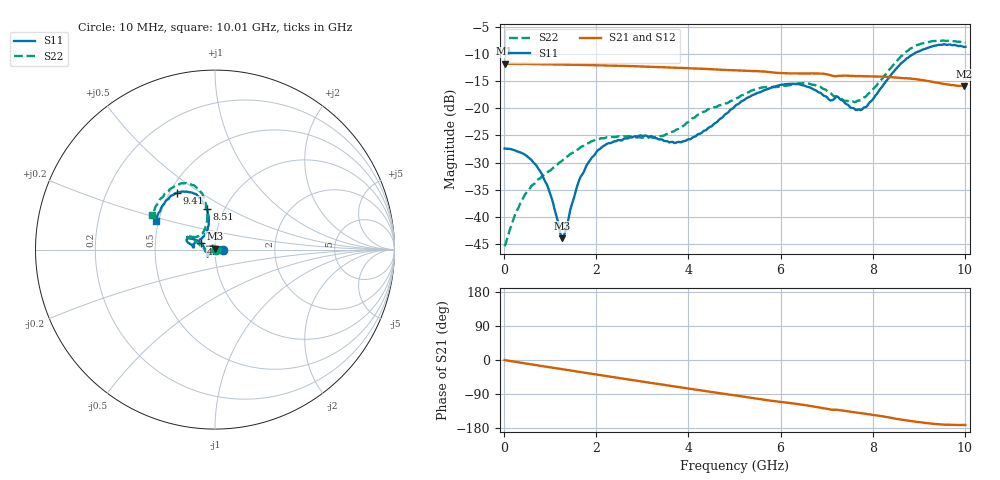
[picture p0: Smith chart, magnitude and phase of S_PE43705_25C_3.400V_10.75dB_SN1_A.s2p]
! Device ID: PE43705
! Serial: 1
! Insertion: A
! Impedance: 50 ohm
! Temp: 25C
! VDD: 3.400V
! Attenuation Step: 10.75dB
#  Hz  S  RI  R  50
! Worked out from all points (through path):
!   401 points, 10 MHz to 10.01 GHz, reference 50 ohm
!   highest |S21| = -11.78 dB at 10 MHz (marker M1); lowest = -15.9 dB at 9.985 GHz (marker M2)
!   group delay of S21, straight-line fit = 49.4 ps
!   lowest |S11| = -43.9 dB at 1.26 GHz (marker M3), VSWR 1.01, Z = 49.8 + j0.605 ohm
!   |S11| at or under -10 dB: start of sweep to 8.89 GHz
!   |S22| runs from -45.4 to -7.5 dB; largest |S21 - S12| = 0.0022
!   S11 on the Smith chart (normalised r, x): 10 MHz: 1.09, +0.00; 4.76 GHz: 0.86, +0.06; 8.51 GHz: 0.83, +0.40; 9.41 GHz: 0.54, +0.40; 10.01 GHz: 0.48, +0.18
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1e7  0.0426 4.91e-05  0.2576 -0.00115  0.2578 -0.00105  0.00537 0.000424
3.85e8  0.0374 0.01  0.2531 -0.0326  0.2543 -0.033  0.0028 0.014
7.35e8  0.024 0.0146  0.2468 -0.0629  0.2468 -0.0628  -0.00738 0.0209
9.85e8  0.0116 0.0124  0.2397 -0.0831  0.2397 -0.083  -0.0173 0.0203
1.26e9  -0.00196 0.00607  0.2301 -0.1037  0.2302 -0.1036  -0.0283 0.0167
1.335e9  -0.00646 0.00385  0.2272 -0.1092  0.2273 -0.1092  -0.0318 0.0151
1.685e9  -0.0228 -0.00868  0.2117 -0.1338  0.2117 -0.1338  -0.044 0.0066
2.235e9  -0.0371 -0.0292  0.182 -0.1678  0.1821 -0.1676  -0.0537 -0.00743
3.36e9  -0.0405 -0.0322  0.1062 -0.2142  0.1064 -0.2139  -0.0544 -0.00354
3.985e9  -0.0513 -0.00501  0.0599 -0.226  0.0601 -0.2258  -0.073 0.0149
4.76e9  -0.077 0.0345  0.004 -0.2257  0.00433 -0.2256  -0.1008 0.0431
5.01e9  -0.0934 0.0469  -0.0133 -0.2229  -0.0131 -0.223  -0.1118 0.05
5.985e9  -0.1517 0.0616  -0.0734 -0.1979  -0.0726 -0.198  -0.1418 0.0699
6.685e9  -0.1469 0.036  -0.1111 -0.177  -0.111 -0.1772  -0.1492 0.0696
7.385e9  -0.1054 0.041  -0.1389 -0.1433  -0.1385 -0.1433  -0.0882 0.0766
7.71e9  -0.0672 0.0706  -0.1506 -0.1277  -0.1498 -0.128  -0.0645 0.0985
8.36e9  -0.0363 0.1913  -0.1711 -0.0917  -0.1704 -0.0921  -0.0454 0.2229
8.51e9  -0.0465 0.2267  -0.1737 -0.0801  -0.1728 -0.0815  -0.0535 0.2622
8.935e9  -0.1038 0.3085  -0.1773 -0.0544  -0.1764 -0.0536  -0.119 0.3584
9.41e9  -0.2129 0.3167  -0.169 -0.0314  -0.1684 -0.0315  -0.2181 0.3595
9.985e9  -0.3244 0.1688  -0.1578 -0.024  -0.1585 -0.0242  -0.3425 0.2062
1.001e10  -0.3312 0.1597  -0.1581 -0.024  -0.159 -0.0247  -0.3499 0.1951
